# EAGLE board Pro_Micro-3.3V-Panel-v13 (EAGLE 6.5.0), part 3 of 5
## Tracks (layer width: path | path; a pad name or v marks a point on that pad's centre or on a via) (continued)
D223  (via drill 0.25)
  Top 0.203: U36.28 111.28,90.4 112.1,90.4 112.67,89.83 112.67,83.19 112.69,83.17 v112.69,81.78
  Bottom 0.203: JP70.2 102.44,81.46 112.37,81.46 v112.69,81.78
D224  (via drill 0.25)
  Top 0.203: 105.18,91.08 105,90.91 105,90.23 v104.75,89.98
  Bottom 0.203: v104.75,89.98 105.92,91.15 105.92,91.95 103.12,94.74 103.12,97.21 102.53,97.8 101.58,97.8 101.23,98.15 101.23,100.74 101.74,101.24 102.45,101.24 103.12,101.92 103.12,104.28 103.12,104.29 102.55,104.87 101.35,104.87 100.85,104.36 100.85,101.56 99.57,100.28 JP70.8
D225  (via drill 0.25)
  Top 0.203: 104.83,91.43 104.32,90.92 v104.29,90.92
  Bottom 0.203: JP70.7 100.84,95.76 100.84,93.98 101.35,93.47 101.35,92.08 102.5,90.92 v104.29,90.92
D226  (via drill 0.25)
  Top 0.203: 108.85,90.73 109.9,89.69 v109.9,89.28
  Bottom 0.203: JP70.6 100.84,93.22 100.84,91.24 101.22,90.86 101.22,88.47 101.71,87.97 101.71,85.78 102.19,85.31 107.23,85.31 108.88,86.97 108.88,87.62 109.9,88.64 v109.9,89.28
D227  (via drill 0.25)
  Top 0.203: 110.94,92.83 111.57,92.19 v111.93,92.19
  Bottom 0.203: JP70.5 100.84,90.68 100.84,88.9 100.8,88.86 100.8,88.28 101.29,87.78 101.29,85.58 102.06,84.82 107.35,84.82 109.3,86.76 109.3,87.38 109.31,87.38 110,88.07 110.55,88.07 111.16,88.68 111.16,89.21 110.41,89.96 109.43,89.96 109.14,90.25 109.14,91.08 109.71,91.65 111.38,91.65 v111.93,92.19
D228  (via drill 0.25)
  Top 0.203: v109.86,90.81 109.86,91.11 v109.86,90.81 | U36.27 109.86,91.12 v109.86,90.81
  Bottom 0.203: v109.86,90.81 110.31,90.81 111.67,89.44 111.67,88.54 110.79,87.67 110.17,87.67 109.71,87.21 109.71,86.54 107.47,84.3 101.83,84.3 100.81,85.32 100.81,87.59 99.57,88.83 JP70.4
D229  (via drill 0.25)
  Top 0.203: JP70.3 100.84,88.14 100.84,93.8 v101.53,94.49 | v102,104.1 102,104.06 102.21,103.84 102.21,103 102.47,102.73 104.24,102.73 104.49,102.98 104.96,102.98 105.39,102.55 105.39,101.96 105.14,101.71 105.14,101.03 105.33,100.85 107.01,100.85 107.01,100.83 107.39,100.45 108.02,100.45 108.12,100.34 108.12,99.59 107.54,99 106.84,99 106.54,99.3 106.36,99.3 106.22,99.16 106.22,98.94 U36.1 106.22,98.94
  Bottom 0.203: v102,104.1 101.96,104.1 101.3,103.44 101.3,101.41 100.84,100.95 100.84,96.65 101.53,95.96 v101.53,94.49
D230
  Top 0.203: JP69.12 114.81,82.47 113.56,83.72 113.56,90.22 112.54,91.24 111.83,91.24 U36.30
D234  (via drill 0.25)
  Top 0.203: R106.1 101.09,83.22 101.09,85.34 101.25,85.5 101.25,91.85 v102.01,92.62 | 103.79,96.49 103.25,97.03 v102.36,97.03
  Bottom 0.203: v102.36,97.03 102.36,92.97 v102.01,92.62
D+  (via drill 0.25)
  Top 0.203: v20.8,36.3 21.59,35.51 21.59,33.78 21.15,33.34 R5.1 | U3.4 13.58,24.39 13.58,26.18 v13.28,26.47
  Bottom 0.203: v20.8,36.3 20.95,36.14 20.95,29.94 19.31,28.3 19.31,26.73 17.77,25.2 17.77,25.18 14.57,25.18 v13.28,26.47
D+1  (via drill 0.25)
  Top 0.203: v39.09,36.3 39.88,35.51 39.88,33.78 39.44,33.34 R10.1 | U4.4 31.87,24.39 31.87,26.18 v31.57,26.47
  Bottom 0.203: v39.09,36.3 39.24,36.14 39.24,29.94 37.6,28.3 37.6,26.73 36.06,25.2 36.06,25.18 32.86,25.18 v31.57,26.47
D+2  (via drill 0.25)
  Top 0.203: v57.38,36.3 58.17,35.51 58.17,33.78 57.73,33.34 R17.1 | U6.4 50.16,24.39 50.16,26.18 v49.86,26.47
  Bottom 0.203: v57.38,36.3 57.53,36.14 57.53,29.94 55.88,28.3 55.88,26.73 54.35,25.2 54.35,25.18 51.15,25.18 v49.86,26.47
D+3  (via drill 0.25)
  Top 0.203: v75.67,36.3 76.45,35.51 76.45,33.78 76.02,33.34 R23.1 | U8.4 68.44,24.39 68.44,26.18 v68.15,26.47
  Bottom 0.203: v75.67,36.3 75.82,36.14 75.82,29.94 74.17,28.3 74.17,26.73 72.64,25.2 72.64,25.18 69.44,25.18 v68.15,26.47
D+4  (via drill 0.25)
  Top 0.203: v93.95,36.3 94.74,35.51 94.74,33.78 94.31,33.34 R29.1 | U10.4 86.73,24.39 86.73,26.18 v86.44,26.47
  Bottom 0.203: v93.95,36.3 94.11,36.14 94.11,29.94 92.46,28.3 92.46,26.73 90.92,25.2 90.92,25.18 87.73,25.18 v86.44,26.47
D+5  (via drill 0.25)
  Top 0.203: v112.24,36.3 113.03,35.51 113.03,33.78 112.59,33.34 R35.1 | U12.4 105.02,24.39 105.02,26.18 v104.72,26.47
  Bottom 0.203: v112.24,36.3 112.39,36.14 112.39,29.94 110.75,28.3 110.75,26.73 109.21,25.2 109.21,25.18 106.02,25.18 v104.72,26.47
D+6  (via drill 0.25)
  Top 0.203: v20.8,73.13 21.59,72.34 21.59,70.61 21.15,70.17 R41.1 | U14.4 13.58,61.22 13.58,63.01 v13.28,63.3
  Bottom 0.203: v20.8,73.13 20.95,72.97 20.95,66.77 19.31,65.13 19.31,63.56 17.77,62.03 17.77,62.01 14.57,62.01 v13.28,63.3
D+7  (via drill 0.25)
  Top 0.203: v39.09,73.13 39.88,72.34 39.88,70.61 39.44,70.17 R47.1 | U16.4 31.87,61.22 31.87,63.01 v31.57,63.3
  Bottom 0.203: v39.09,73.13 39.24,72.97 39.24,66.77 37.6,65.13 37.6,63.56 36.06,62.03 36.06,62.01 32.86,62.01 v31.57,63.3
D+8  (via drill 0.25)
  Top 0.203: v57.38,73.13 58.17,72.34 58.17,70.61 57.73,70.17 R53.1 | U18.4 50.16,61.22 50.16,63.01 v49.86,63.3
  Bottom 0.203: v57.38,73.13 57.53,72.97 57.53,66.77 55.88,65.13 55.88,63.56 54.35,62.03 54.35,62.01 51.15,62.01 v49.86,63.3
D+9  (via drill 0.25)
  Top 0.203: v75.67,73.13 76.45,72.34 76.45,70.61 76.02,70.17 R59.1 | U20.4 68.44,61.22 68.44,63.01 v68.15,63.3
  Bottom 0.203: v75.67,73.13 75.82,72.97 75.82,66.77 74.17,65.13 74.17,63.56 72.64,62.03 72.64,62.01 69.44,62.01 v68.15,63.3
D+10  (via drill 0.25)
  Top 0.203: v93.95,73.13 94.74,72.34 94.74,70.61 94.31,70.17 R65.1 | U22.4 86.73,61.22 86.73,63.01 v86.44,63.3
  Bottom 0.203: v93.95,73.13 94.11,72.97 94.11,66.77 92.46,65.13 92.46,63.56 90.92,62.03 90.92,62.01 87.73,62.01 v86.44,63.3
D+11  (via drill 0.25)
  Top 0.203: v112.24,73.13 113.03,72.34 113.03,70.61 112.59,70.17 R71.1 | U24.4 105.02,61.22 105.02,63.01 v104.72,63.3
  Bottom 0.203: v112.24,73.13 112.39,72.97 112.39,66.77 110.75,65.13 110.75,63.56 109.21,62.03 109.21,62.01 106.02,62.01 v104.72,63.3
D+12  (via drill 0.25)
  Top 0.203: v20.8,109.96 21.59,109.17 21.59,107.44 21.15,107 R77.1 | U26.4 13.58,98.05 13.58,99.83 v13.28,100.13
  Bottom 0.203: v20.8,109.96 20.95,109.8 20.95,103.6 19.31,101.96 19.31,100.39 17.77,98.86 17.77,98.84 14.57,98.84 v13.28,100.13
D+13  (via drill 0.25)
  Top 0.203: v39.09,109.96 39.88,109.17 39.88,107.44 39.44,107 R83.1 | U28.4 31.87,98.05 31.87,99.83 v31.57,100.13
  Bottom 0.203: v39.09,109.96 39.24,109.8 39.24,103.6 37.6,101.96 37.6,100.39 36.06,98.86 36.06,98.84 32.86,98.84 v31.57,100.13
D+14  (via drill 0.25)
  Top 0.203: v57.38,109.96 58.17,109.17 58.17,107.44 57.73,107 R89.1 | U30.4 50.16,98.05 50.16,99.83 v49.86,100.13
  Bottom 0.203: v57.38,109.96 57.53,109.8 57.53,103.6 55.88,101.96 55.88,100.39 54.35,98.86 54.35,98.84 51.15,98.84 v49.86,100.13
D+15  (via drill 0.25)
  Top 0.203: v75.67,109.96 76.45,109.17 76.45,107.44 76.02,107 R95.1 | U32.4 68.44,98.05 68.44,99.83 v68.15,100.13
  Bottom 0.203: v75.67,109.96 75.82,109.8 75.82,103.6 74.17,101.96 74.17,100.39 72.64,98.86 72.64,98.84 69.44,98.84 v68.15,100.13
D+16  (via drill 0.25)
  Top 0.203: v93.95,109.96 94.74,109.17 94.74,107.44 94.31,107 R101.1 | U34.4 86.73,98.05 86.73,99.83 v86.44,100.13
  Bottom 0.203: v93.95,109.96 94.11,109.8 94.11,103.6 92.46,101.96 92.46,100.39 90.92,98.86 90.92,98.84 87.73,98.84 v86.44,100.13
D+17  (via drill 0.25)
  Top 0.203: v112.24,109.96 113.03,109.17 113.03,107.44 112.59,107 R107.1 | U36.4 105.02,98.05 105.02,99.83 v104.72,100.13
  Bottom 0.203: v112.24,109.96 112.39,109.8 112.39,103.6 110.75,101.96 110.75,100.39 109.21,98.86 109.21,98.84 106.02,98.84 v104.72,100.13
D-  (via drill 0.25)
  Top 0.203: 20.41,35.12 R7.1 20.32,34.89 20.32,35.56 19.96,35.92 v19.96,37.08 | v14.25,26.5 13.99,26.25 13.99,24.67 14.1,24.57
  Bottom 0.203: v19.96,37.08 21.08,37.08 21.46,36.7 21.46,29.77 19.76,28.07 19.76,26.53 17.98,24.75 14.43,24.75 13.44,25.75 13.04,25.75 13.03,25.74 12.58,26.2 12.58,26.86 12.93,27.21 13.54,27.21 v14.25,26.5
D-1  (via drill 0.25)
  Top 0.203: 38.7,35.12 R12.1 38.61,34.89 38.61,35.56 38.25,35.92 v38.25,37.08 | v32.53,26.5 32.28,26.25 32.28,24.67 32.38,24.57
  Bottom 0.203: v38.25,37.08 39.37,37.08 39.75,36.7 39.75,29.77 38.05,28.07 38.05,26.53 36.27,24.75 32.72,24.75 31.73,25.75 31.33,25.75 31.32,25.74 30.87,26.2 30.87,26.86 31.22,27.21 31.83,27.21 v32.53,26.5
D-2  (via drill 0.25)
  Top 0.203: 56.98,35.12 R18.1 56.9,34.89 56.9,35.56 56.54,35.92 v56.54,37.08 | v50.82,26.5 50.57,26.25 50.57,24.67 50.67,24.57
  Bottom 0.203: v56.54,37.08 57.66,37.08 58.04,36.7 58.04,29.77 56.34,28.07 56.34,26.53 54.56,24.75 51.01,24.75 50.02,25.75 49.62,25.75 49.61,25.74 49.15,26.2 49.15,26.86 49.51,27.21 50.11,27.21 v50.82,26.5
D-3  (via drill 0.25)
  Top 0.203: 75.27,35.12 R24.1 75.18,34.89 75.18,35.56 74.83,35.92 v74.83,37.08 | v69.11,26.5 68.86,26.25 68.86,24.67 68.96,24.57
  Bottom 0.203: v74.83,37.08 75.95,37.08 76.33,36.7 76.33,29.77 74.62,28.07 74.62,26.53 72.85,24.75 69.3,24.75 68.3,25.75 67.9,25.75 67.9,25.74 67.44,26.2 67.44,26.86 67.79,27.21 68.4,27.21 v69.11,26.5
D-4  (via drill 0.25)
  Top 0.203: 93.56,35.12 R30.1 93.47,34.89 93.47,35.56 93.12,35.92 v93.12,37.08 | v87.4,26.5 87.15,26.25 87.15,24.67 87.25,24.57
  Bottom 0.203: v93.12,37.08 94.23,37.08 94.61,36.7 94.61,29.77 92.91,28.07 92.91,26.53 91.14,24.75 87.58,24.75 86.59,25.75 86.19,25.75 86.19,25.74 85.73,26.2 85.73,26.86 86.08,27.21 86.69,27.21 v87.4,26.5
D-5  (via drill 0.25)
  Top 0.203: 111.85,35.12 R36.1 111.76,34.89 111.76,35.56 111.4,35.92 v111.4,37.08 | v105.69,26.5 105.44,26.25 105.44,24.67 105.54,24.57
  Bottom 0.203: v111.4,37.08 112.52,37.08 112.9,36.7 112.9,29.77 111.2,28.07 111.2,26.53 109.42,24.75 105.87,24.75 104.88,25.75 104.48,25.75 104.47,25.74 104.02,26.2 104.02,26.86 104.37,27.21 104.98,27.21 v105.69,26.5
D-6  (via drill 0.25)
  Top 0.203: 20.41,71.95 R42.1 20.32,71.72 20.32,72.39 19.96,72.75 v19.96,73.91 | v14.25,63.34 13.99,63.08 13.99,61.5 14.1,61.4
  Bottom 0.203: v19.96,73.91 21.08,73.91 21.46,73.53 21.46,66.6 19.76,64.9 19.76,63.36 17.98,61.59 14.43,61.59 13.44,62.58 13.04,62.58 13.03,62.57 12.58,63.02 12.58,63.69 12.93,64.04 13.54,64.04 v14.25,63.34
D-7  (via drill 0.25)
  Top 0.203: 38.7,71.95 R48.1 38.61,71.72 38.61,72.39 38.25,72.75 v38.25,73.91 | v32.53,63.34 32.28,63.08 32.28,61.5 32.38,61.4
  Bottom 0.203: v38.25,73.91 39.37,73.91 39.75,73.53 39.75,66.6 38.05,64.9 38.05,63.36 36.27,61.59 32.72,61.59 31.73,62.58 31.33,62.58 31.32,62.57 30.87,63.02 30.87,63.69 31.22,64.04 31.83,64.04 v32.53,63.34
D-8  (via drill 0.25)
  Top 0.203: 56.98,71.95 R54.1 56.9,71.72 56.9,72.39 56.54,72.75 v56.54,73.91 | v50.82,63.34 50.57,63.08 50.57,61.5 50.67,61.4
  Bottom 0.203: v56.54,73.91 57.66,73.91 58.04,73.53 58.04,66.6 56.34,64.9 56.34,63.36 54.56,61.59 51.01,61.59 50.02,62.58 49.62,62.58 49.61,62.57 49.15,63.02 49.15,63.69 49.51,64.04 50.11,64.04 v50.82,63.34
D-9  (via drill 0.25)
  Top 0.203: 75.27,71.95 R60.1 75.18,71.72 75.18,72.39 74.83,72.75 v74.83,73.91 | v69.11,63.34 68.86,63.08 68.86,61.5 68.96,61.4
  Bottom 0.203: v74.83,73.91 75.95,73.91 76.33,73.53 76.33,66.6 74.62,64.9 74.62,63.36 72.85,61.59 69.3,61.59 68.3,62.58 67.9,62.58 67.9,62.57 67.44,63.02 67.44,63.69 67.79,64.04 68.4,64.04 v69.11,63.34
D-10  (via drill 0.25)
  Top 0.203: 93.56,71.95 R66.1 93.47,71.72 93.47,72.39 93.12,72.75 v93.12,73.91 | v87.4,63.34 87.15,63.08 87.15,61.5 87.25,61.4
  Bottom 0.203: v93.12,73.91 94.23,73.91 94.61,73.53 94.61,66.6 92.91,64.9 92.91,63.36 91.14,61.59 87.58,61.59 86.59,62.58 86.19,62.58 86.19,62.57 85.73,63.02 85.73,63.69 86.08,64.04 86.69,64.04 v87.4,63.34
D-11  (via drill 0.25)
  Top 0.203: 111.85,71.95 R72.1 111.76,71.72 111.76,72.39 111.4,72.75 v111.4,73.91 | v105.69,63.34 105.44,63.08 105.44,61.5 105.54,61.4
  Bottom 0.203: v111.4,73.91 112.52,73.91 112.9,73.53 112.9,66.6 111.2,64.9 111.2,63.36 109.42,61.59 105.87,61.59 104.88,62.58 104.48,62.58 104.47,62.57 104.02,63.02 104.02,63.69 104.37,64.04 104.98,64.04 v105.69,63.34
D-12  (via drill 0.25)
  Top 0.203: 20.41,108.78 R78.1 20.32,108.55 20.32,109.22 19.96,109.58 v19.96,110.74 | v14.25,100.17 13.99,99.91 13.99,98.33 14.1,98.23
  Bottom 0.203: v19.96,110.74 21.08,110.74 21.46,110.36 21.46,103.43 19.76,101.73 19.76,100.19 17.98,98.42 14.43,98.42 13.44,99.41 13.04,99.41 13.03,99.4 12.58,99.86 12.58,100.52 12.93,100.87 13.54,100.87 v14.25,100.17
D-13  (via drill 0.25)
  Top 0.203: 38.7,108.78 R84.1 38.61,108.55 38.61,109.22 38.25,109.58 v38.25,110.74 | v32.53,100.17 32.28,99.91 32.28,98.33 32.38,98.23
  Bottom 0.203: v38.25,110.74 39.37,110.74 39.75,110.36 39.75,103.43 38.05,101.73 38.05,100.19 36.27,98.42 32.72,98.42 31.73,99.41 31.33,99.41 31.32,99.4 30.87,99.86 30.87,100.52 31.22,100.87 31.83,100.87 v32.53,100.17
D-14  (via drill 0.25)
  Top 0.203: 56.98,108.78 R90.1 56.9,108.55 56.9,109.22 56.54,109.58 v56.54,110.74 | v50.82,100.17 50.57,99.91 50.57,98.33 50.67,98.23
  Bottom 0.203: v56.54,110.74 57.66,110.74 58.04,110.36 58.04,103.43 56.34,101.73 56.34,100.19 54.56,98.42 51.01,98.42 50.02,99.41 49.62,99.41 49.61,99.4 49.15,99.86 49.15,100.52 49.51,100.87 50.11,100.87 v50.82,100.17
D-15  (via drill 0.25)
  Top 0.203: 75.27,108.78 R96.1 75.18,108.55 75.18,109.22 74.83,109.58 v74.83,110.74 | v69.11,100.17 68.86,99.91 68.86,98.33 68.96,98.23
  Bottom 0.203: v74.83,110.74 75.95,110.74 76.33,110.36 76.33,103.43 74.62,101.73 74.62,100.19 72.85,98.42 69.3,98.42 68.3,99.41 67.9,99.41 67.9,99.4 67.44,99.86 67.44,100.52 67.79,100.87 68.4,100.87 v69.11,100.17
D-16  (via drill 0.25)
  Top 0.203: 93.56,108.78 R102.1 93.47,108.55 93.47,109.22 93.12,109.58 v93.12,110.74 | v87.4,100.17 87.15,99.91 87.15,98.33 87.25,98.23
  Bottom 0.203: v93.12,110.74 94.23,110.74 94.61,110.36 94.61,103.43 92.91,101.73 92.91,100.19 91.14,98.42 87.58,98.42 86.59,99.41 86.19,99.41 86.19,99.4 85.73,99.86 85.73,100.52 86.08,100.87 86.69,100.87 v87.4,100.17
D-17  (via drill 0.25)
  Top 0.203: 111.85,108.78 R108.1 111.76,108.55 111.76,109.22 111.4,109.58 v111.4,110.74 | v105.69,100.17 105.44,99.91 105.44,98.33 105.54,98.23
  Bottom 0.203: v111.4,110.74 112.52,110.74 112.9,110.36 112.9,103.43 111.2,101.73 111.2,100.19 109.42,98.42 105.87,98.42 104.88,99.41 104.48,99.41 104.47,99.4 104.02,99.86 104.02,100.52 104.37,100.87 104.98,100.87 v105.69,100.17
GND  (via drill 0.25)
  Top 0.203: v20.57,19.48 | U3.33 20.5,19.56 20.83,19.56 | C3.1 20.07,14.33 | 12.34,18.82 12.22,18.82 11.76,18.36 11.52,18.36 11.05,17.89 11.05,17.32 11.32,17.06 C10.2 11.49,15.41 12.12,14.78 12.12,13.64 12.99,12.77 C4.2 | 16.71,16.38 16.76,16.33 16.76,15.93 | 18.2,13.84 arc-21 v19.05,13.31 | 12.24,27.31 C13.C 12.56,26.67 C5.1 12.56,24.71 13.4,23.87
  Top 0.406: X1.GND1 14.45,37.34 14.48,37.34
  Bottom 0.203: JP7.10 9.25,32.11 v10.2,32.11
  other vias: 15.99,9.86 21.72,25.53 18.76,28.77 20.74,22.7 17.74,26.5 13.25,28.57 23.94,38.23 15.44,32.56 22.26,29.71 13.68,37.82 10.37,9.85 12.46,13.81 13.28,31.04 16.41,13.92
  pour Top (isolate 0.203): 6.86,39.88 24.64,39.88 24.64,6.86 6.86,6.86
  pour Bottom (isolate 0.203): 6.86,39.88 24.64,39.88 24.64,6.86 6.86,6.86
GND1  (via drill 0.25)
  Top 0.203: v38.86,19.48 | U4.33 38.79,19.56 39.12,19.56 | C9.1 38.35,14.33 | 30.63,18.82 30.51,18.82 30.05,18.36 29.81,18.36 29.34,17.89 29.34,17.32 29.6,17.06 C7.2 29.78,15.41 30.41,14.78 30.41,13.64 31.28,12.77 C15.2 | 35,16.38 35.05,16.33 35.05,15.93 | 36.49,13.84 arc-21 v37.33,13.31 | 30.53,27.31 C8.C 30.85,26.67 C16.1 30.85,24.71 31.69,23.87
  Top 0.406: X2.GND1 32.74,37.34 32.77,37.34
  Bottom 0.203: JP4.10 27.54,32.11 v28.49,32.11
  other vias: 34.27,9.86 40.01,25.53 37.05,28.77 39.03,22.7 36.03,26.5 31.54,28.57 42.23,38.23 33.73,32.56 40.54,29.71 31.97,37.82 28.65,9.85 30.75,13.81 31.57,31.04 34.7,13.92
  pour Top (isolate 0.203): 25.15,39.88 42.93,39.88 42.93,6.86 25.15,6.86
  pour Bottom (isolate 0.203): 25.15,39.88 42.93,39.88 42.93,6.86 25.15,6.86
GND2  (via drill 0.25)
  Top 0.203: v57.15,19.48 | U6.33 57.08,19.56 57.4,19.56 | C21.1 56.64,14.33 | 48.92,18.82 48.79,18.82 48.33,18.36 48.09,18.36 47.63,17.89 47.63,17.32 47.89,17.06 C18.2 48.06,15.41 48.07,15.41 48.7,14.78 48.7,13.64 49.57,12.77 C25.2 | 53.29,16.38 53.34,16.33 53.34,15.93 | 54.77,13.84 arc-21 v55.62,13.31 | 48.81,27.31 C20.C 49.14,26.67 C26.1 49.14,24.71 49.98,23.87
  Top 0.406: X3.GND1 51.02,37.34 51.05,37.34
  Bottom 0.203: JP10.10 45.83,32.11 v46.77,32.11
  other vias: 52.56,9.86 58.29,25.53 55.34,28.77 57.32,22.7 54.32,26.5 49.82,28.57 60.52,38.23 52.02,32.56 58.83,29.71 50.25,37.82 46.94,9.85 49.03,13.81 49.86,31.04 52.99,13.92
  pour Top (isolate 0.203): 43.43,39.88 61.21,39.88 61.21,6.86 43.43,6.86
  pour Bottom (isolate 0.203): 43.43,39.88 61.21,39.88 61.21,6.86 43.43,6.86
GND3  (via drill 0.25)
  Top 0.203: v75.43,19.48 v75.44,19.48 | U8.33 75.37,19.56 75.69,19.56 | C30.1 74.93,14.33 | 67.21,18.82 67.08,18.82 66.62,18.36 66.38,18.36 65.92,17.89 65.92,17.32 66.18,17.06 C28.2 66.35,15.41 66.36,15.41 66.98,14.78 66.98,13.64 67.86,12.77 C34.2 | 71.58,16.38 71.63,16.33 71.63,15.93 | 73.06,13.84 arc-21 v73.91,13.31 | 67.1,27.31 C29.C 67.43,26.67 C35.1 67.43,24.71 68.26,23.87
  Top 0.406: X4.GND1 69.31,37.34 69.34,37.34
  Bottom 0.203: JP14.10 64.11,32.11 v65.06,32.11
  other vias: 70.85,9.86 76.58,25.53 73.62,28.77 75.6,22.7 72.61,26.5 68.11,28.57 78.8,38.23 70.3,32.56 77.12,29.71 68.54,37.82 65.23,9.85 67.32,13.81 68.15,31.04 71.28,13.92
  pour Top (isolate 0.203): 61.72,39.88 79.5,39.88 79.5,6.86 61.72,6.86
  pour Bottom (isolate 0.203): 61.72,39.88 79.5,39.88 79.5,6.86 61.72,6.86
GND4  (via drill 0.25)
  Top 0.203: v93.72,19.48 v93.73,19.48 | U10.33 93.66,19.56 93.98,19.56 | C39.1 93.22,14.33 | 85.5,18.82 85.37,18.82 84.91,18.36 84.67,18.36 84.21,17.89 84.21,17.32 84.47,17.06 C37.2 84.64,15.41 85.27,14.78 85.27,13.64 86.14,12.77 C43.2 | 89.86,16.38 89.92,16.33 89.92,15.93 | 91.35,13.84 arc-21 v92.2,13.31 | 85.39,27.31 C38.C 85.71,26.67 C44.1 85.71,24.71 86.55,23.87
  Top 0.406: X5.GND1 87.6,37.34 87.63,37.34
  Bottom 0.203: JP18.10 82.4,32.11 v83.35,32.11
  other vias: 89.14,9.86 94.87,25.53 91.91,28.77 93.89,22.7 90.89,26.5 86.4,28.57 97.09,38.23 88.59,32.56 95.41,29.71 86.83,37.82 83.52,9.85 85.61,13.81 86.44,31.04 89.57,13.92
  pour Top (isolate 0.203): 80.01,39.88 97.79,39.88 97.79,6.86 80.01,6.86
  pour Bottom (isolate 0.203): 80.01,39.88 97.79,39.88 97.79,6.86 80.01,6.86
GND5  (via drill 0.25)
  Top 0.203: v112.01,19.48 | U12.33 111.94,19.56 112.27,19.56 | C48.1 111.51,14.33 | 103.78,18.82 103.66,18.82 103.2,18.36 102.96,18.36 102.49,17.89 102.49,17.32 102.76,17.06 C46.2 102.93,15.41 103.56,14.78 103.56,13.64 104.43,12.77 C52.2 | 108.15,16.38 108.2,16.33 108.2,15.93 | 109.64,13.84 arc-21 v110.48,13.31 | 103.68,27.31 C47.C 104,26.67 C53.1 104,24.71 104.84,23.87
  Top 0.406: X6.GND1 105.89,37.34 105.92,37.34
  Bottom 0.203: JP22.10 100.69,32.11 v101.64,32.11
  other vias: 107.43,9.86 113.16,25.53 110.2,28.77 112.18,22.7 109.18,26.5 104.69,28.57 115.38,38.23 106.88,32.56 113.7,29.71 105.12,37.82 101.81,9.85 103.9,13.81 104.72,31.04 107.85,13.92
  pour Top (isolate 0.203): 98.3,39.88 116.08,39.88 116.08,6.86 98.3,6.86
  pour Bottom (isolate 0.203): 98.3,39.88 116.08,39.88 116.08,6.86 98.3,6.86
GND6  (via drill 0.25)
  Top 0.203: v20.57,56.31 | U14.33 20.5,56.39 20.83,56.39 | C57.1 20.07,51.16 | 12.34,55.65 12.22,55.65 11.76,55.19 11.52,55.19 11.05,54.72 11.05,54.15 11.32,53.89 C55.2 11.49,52.24 12.12,51.61 12.12,50.47 12.99,49.59 C61.2 | 16.71,53.21 16.76,53.16 16.76,52.76 | 18.2,50.67 arc-21 v19.05,50.15 | 12.24,64.14 C56.C 12.56,63.5 C62.1 12.56,61.54 13.4,60.7
  Top 0.406: X7.GND1 14.45,74.17 14.48,74.17
  Bottom 0.203: JP26.10 9.25,68.94 v10.2,68.94
  other vias: 15.99,46.69 21.72,62.36 18.76,65.6 20.74,59.53 17.74,63.33 13.25,65.4 23.94,75.06 15.44,69.39 22.26,66.54 13.68,74.65 10.37,46.68 12.46,50.64 13.28,67.87 16.41,50.75
  pour Top (isolate 0.203): 6.86,76.71 24.64,76.71 24.64,43.69 6.86,43.69
  pour Bottom (isolate 0.203): 6.86,76.71 24.64,76.71 24.64,43.69 6.86,43.69
GND7  (via drill 0.25)
  Top 0.203: v38.86,56.31 | U16.33 38.79,56.39 39.12,56.39 | C66.1 38.35,51.16 | 30.63,55.65 30.51,55.65 30.05,55.19 29.81,55.19 29.34,54.72 29.34,54.15 29.6,53.89 C64.2 29.78,52.24 30.41,51.61 30.41,50.47 31.28,49.59 C70.2 | 35,53.21 35.05,53.16 35.05,52.76 | 36.49,50.67 arc-21 v37.33,50.15 | 30.53,64.14 C65.C 30.85,63.5 C71.1 30.85,61.54 31.69,60.7
  Top 0.406: X8.GND1 32.74,74.17 32.77,74.17
  Bottom 0.203: JP30.10 27.54,68.94 v28.49,68.94
  other vias: 34.27,46.69 40.01,62.36 37.05,65.6 39.03,59.53 36.03,63.33 31.54,65.4 42.23,75.06 33.73,69.39 40.54,66.54 31.97,74.65 28.65,46.68 30.75,50.64 31.57,67.87 34.7,50.75
  pour Top (isolate 0.203): 25.15,76.71 42.93,76.71 42.93,43.69 25.15,43.69
  pour Bottom (isolate 0.203): 25.15,76.71 42.93,76.71 42.93,43.69 25.15,43.69
GND8  (via drill 0.25)
  Top 0.203: v57.15,56.31 | U18.33 57.08,56.39 57.4,56.39 | C75.1 56.64,51.16 | 48.92,55.65 48.79,55.65 48.33,55.19 48.09,55.19 47.63,54.72 47.63,54.15 47.89,53.89 C73.2 48.06,52.24 48.07,52.24 48.7,51.61 48.7,50.47 49.57,49.59 C79.2 | 53.29,53.21 53.34,53.16 53.34,52.76 | 54.77,50.67 arc-21 v55.62,50.15 | 48.81,64.14 C74.C 49.14,63.5 C80.1 49.14,61.54 49.98,60.7
  Top 0.406: X9.GND1 51.02,74.17 51.05,74.17
  Bottom 0.203: JP34.10 45.83,68.94 v46.77,68.94
  other vias: 52.56,46.69 58.29,62.36 55.34,65.6 57.32,59.53 54.32,63.33 49.82,65.4 60.52,75.06 52.02,69.39 58.83,66.54 50.25,74.65 46.94,46.68 49.03,50.64 49.86,67.87 52.99,50.75
  pour Top (isolate 0.203): 43.43,76.71 61.21,76.71 61.21,43.69 43.43,43.69
  pour Bottom (isolate 0.203): 43.43,76.71 61.21,76.71 61.21,43.69 43.43,43.69
GND9  (via drill 0.25)
  Top 0.203: v75.43,56.31 v75.44,56.31 | U20.33 75.37,56.39 75.69,56.39 | C84.1 74.93,51.16 | 67.21,55.65 67.08,55.65 66.62,55.19 66.38,55.19 65.92,54.72 65.92,54.15 66.18,53.89 C82.2 66.35,52.24 66.36,52.24 66.98,51.61 66.98,50.47 67.86,49.59 C88.2 | 71.58,53.21 71.63,53.16 71.63,52.76 | 73.06,50.67 arc-21 v73.91,50.15 | 67.1,64.14 C83.C 67.43,63.5 C89.1 67.43,61.54 68.26,60.7
  Top 0.406: X10.GND1 69.31,74.17 69.34,74.17
  Bottom 0.203: JP38.10 64.11,68.94 v65.06,68.94
  other vias: 70.85,46.69 76.58,62.36 73.62,65.6 75.6,59.53 72.61,63.33 68.11,65.4 78.8,75.06 70.3,69.39 77.12,66.54 68.54,74.65 65.23,46.68 67.32,50.64 68.15,67.87 71.28,50.75
  pour Top (isolate 0.203): 61.72,76.71 79.5,76.71 79.5,43.69 61.72,43.69
  pour Bottom (isolate 0.203): 61.72,76.71 79.5,76.71 79.5,43.69 61.72,43.69
GND10  (via drill 0.25)
  Top 0.203: v93.72,56.31 v93.73,56.31 | U22.33 93.66,56.39 93.98,56.39 | C93.1 93.22,51.16 | 85.5,55.65 85.37,55.65 84.91,55.19 84.67,55.19 84.21,54.72 84.21,54.15 84.47,53.89 C91.2 84.64,52.24 85.27,51.61 85.27,50.47 86.14,49.59 C97.2 | 89.86,53.21 89.92,53.16 89.92,52.76 | 91.35,50.67 arc-21 v92.2,50.15 | 85.39,64.14 C92.C 85.71,63.5 C98.1 85.71,61.54 86.55,60.7
  Top 0.406: X11.GND1 87.6,74.17 87.63,74.17
  Bottom 0.203: JP42.10 82.4,68.94 v83.35,68.94
  other vias: 89.14,46.69 94.87,62.36 91.91,65.6 93.89,59.53 90.89,63.33 86.4,65.4 97.09,75.06 88.59,69.39 95.41,66.54 86.83,74.65 83.52,46.68 85.61,50.64 86.44,67.87 89.57,50.75
  pour Top (isolate 0.203): 80.01,76.71 97.79,76.71 97.79,43.69 80.01,43.69
  pour Bottom (isolate 0.203): 80.01,76.71 97.79,76.71 97.79,43.69 80.01,43.69
GND11  (via drill 0.25)
  Top 0.203: v112.01,56.31 | U24.33 111.94,56.39 112.27,56.39 | C102.1 111.51,51.16 | 103.78,55.65 103.66,55.65 103.2,55.19 102.96,55.19 102.49,54.72 102.49,54.15 102.76,53.89 C100.2 102.93,52.24 103.56,51.61 103.56,50.47 104.43,49.59 C106.2 | 108.15,53.21 108.2,53.16 108.2,52.76 | 109.64,50.67 arc-21 v110.48,50.15 | 103.68,64.14 C101.C 104,63.5 C107.1 104,61.54 104.84,60.7
  Top 0.406: X12.GND1 105.89,74.17 105.92,74.17
  Bottom 0.203: JP46.10 100.69,68.94 v101.64,68.94
  other vias: 107.43,46.69 113.16,62.36 110.2,65.6 112.18,59.53 109.18,63.33 104.69,65.4 115.38,75.06 106.88,69.39 113.7,66.54 105.12,74.65 101.81,46.68 103.9,50.64 104.72,67.87 107.85,50.75
  pour Top (isolate 0.203): 98.3,76.71 116.08,76.71 116.08,43.69 98.3,43.69
  pour Bottom (isolate 0.203): 98.3,76.71 116.08,76.71 116.08,43.69 98.3,43.69
GND12  (via drill 0.25)
  Top 0.203: v20.57,93.14 | U26.33 20.5,93.22 20.83,93.22 | C111.1 20.07,87.99 | 12.34,92.48 12.22,92.48 11.76,92.02 11.52,92.02 11.05,91.55 11.05,90.98 11.32,90.72 C109.2 11.49,89.07 12.12,88.44 12.12,87.3 12.99,86.42 C115.2 | 16.71,90.04 16.76,89.99 16.76,89.59 | 18.2,87.5 arc-21 v19.05,86.97 | 12.24,100.97 C110.C 12.56,100.33 C116.1 12.56,98.37 13.4,97.53
  Top 0.406: X13.GND1 14.45,111 14.48,111
  Bottom 0.203: JP50.10 9.25,105.77 v10.2,105.77
  other vias: 15.99,83.52 21.72,99.19 18.76,102.43 20.74,96.36 17.74,100.16 13.25,102.23 23.94,111.89 15.44,106.22 22.26,103.37 13.68,111.48 10.37,83.51 12.46,87.47 13.28,104.7 16.41,87.58
  pour Top (isolate 0.203): 6.86,113.54 24.64,113.54 24.64,80.52 6.86,80.52
  pour Bottom (isolate 0.203): 6.86,113.54 24.64,113.54 24.64,80.52 6.86,80.52
GND13  (via drill 0.25)
  Top 0.203: v38.86,93.14 | U28.33 38.79,93.22 39.12,93.22 | C120.1 38.35,87.99 | 30.63,92.48 30.51,92.48 30.05,92.02 29.81,92.02 29.34,91.55 29.34,90.98 29.6,90.72 C118.2 29.78,89.07 30.41,88.44 30.41,87.3 31.28,86.42 C124.2 | 35,90.04 35.05,89.99 35.05,89.59 | 36.49,87.5 arc-21 v37.33,86.97 | 30.53,100.97 C119.C 30.85,100.33 C125.1 30.85,98.37 31.69,97.53
  Top 0.406: X14.GND1 32.74,111 32.77,111
  Bottom 0.203: JP54.10 27.54,105.77 v28.49,105.77
  other vias: 34.27,83.52 40.01,99.19 37.05,102.43 39.03,96.36 36.03,100.16 31.54,102.23 42.23,111.89 33.73,106.22 40.54,103.37 31.97,111.48 28.65,83.51 30.75,87.47 31.57,104.7 34.7,87.58
  pour Top (isolate 0.203): 25.15,113.54 42.93,113.54 42.93,80.52 25.15,80.52
  pour Bottom (isolate 0.203): 25.15,113.54 42.93,113.54 42.93,80.52 25.15,80.52
GND14  (via drill 0.25)
  Top 0.203: v57.15,93.14 | U30.33 57.08,93.22 57.4,93.22 | C129.1 56.64,87.99 | 48.92,92.48 48.79,92.48 48.33,92.02 48.09,92.02 47.63,91.55 47.63,90.98 47.89,90.72 C127.2 48.06,89.07 48.07,89.07 48.7,88.44 48.7,87.3 49.57,86.42 C133.2 | 53.29,90.04 53.34,89.99 53.34,89.59 | 54.77,87.5 arc-21 v55.62,86.97 | 48.81,100.97 C128.C 49.14,100.33 C134.1 49.14,98.37 49.98,97.53
  Top 0.406: X15.GND1 51.02,111 51.05,111
  Bottom 0.203: JP58.10 45.83,105.77 v46.77,105.77
  other vias: 52.56,83.52 58.29,99.19 55.34,102.43 57.32,96.36 54.32,100.16 49.82,102.23 60.52,111.89 52.02,106.22 58.83,103.37 50.25,111.48 46.94,83.51 49.03,87.47 49.86,104.7 52.99,87.58
  pour Top (isolate 0.203): 43.43,113.54 61.21,113.54 61.21,80.52 43.43,80.52
  pour Bottom (isolate 0.203): 43.43,113.54 61.21,113.54 61.21,80.52 43.43,80.52
GND15  (via drill 0.25)
  Top 0.203: v75.43,93.14 v75.44,93.14 | U32.33 75.37,93.22 75.69,93.22 | C138.1 74.93,87.99 | 67.21,92.48 67.08,92.48 66.62,92.02 66.38,92.02 65.92,91.55 65.92,90.98 66.18,90.72 C136.2 66.35,89.07 66.36,89.07 66.98,88.44 66.98,87.3 67.86,86.42 C142.2 | 71.58,90.04 71.63,89.99 71.63,89.59 | 73.06,87.5 arc-21 v73.91,86.97 | 67.1,100.97 C137.C 67.43,100.33 C143.1 67.43,98.37 68.26,97.53
  Top 0.406: X16.GND1 69.31,111 69.34,111
  Bottom 0.203: JP62.10 64.11,105.77 v65.06,105.77
  other vias: 70.85,83.52 76.58,99.19 73.62,102.43 75.6,96.36 72.61,100.16 68.11,102.23 78.8,111.89 70.3,106.22 77.12,103.37 68.54,111.48 65.23,83.51 67.32,87.47 68.15,104.7 71.28,87.58
  pour Top (isolate 0.203): 61.72,113.54 79.5,113.54 79.5,80.52 61.72,80.52
  pour Bottom (isolate 0.203): 61.72,113.54 79.5,113.54 79.5,80.52 61.72,80.52
GND16  (via drill 0.25)
  Top 0.203: v93.72,93.14 v93.73,93.14 | U34.33 93.66,93.22 93.98,93.22 | C147.1 93.22,87.99 | 85.5,92.48 85.37,92.48 84.91,92.02 84.67,92.02 84.21,91.55 84.21,90.98 84.47,90.72 C145.2 84.64,89.07 85.27,88.44 85.27,87.3 86.14,86.42 C151.2 | 89.86,90.04 89.92,89.99 89.92,89.59 | 91.35,87.5 arc-21 v92.2,86.97 | 85.39,100.97 C146.C 85.71,100.33 C152.1 85.71,98.37 86.55,97.53
  Top 0.406: X17.GND1 87.6,111 87.63,111
  Bottom 0.203: JP66.10 82.4,105.77 v83.35,105.77
  other vias: 89.14,83.52 94.87,99.19 91.91,102.43 93.89,96.36 90.89,100.16 86.4,102.23 97.09,111.89 88.59,106.22 95.41,103.37 86.83,111.48 83.52,83.51 85.61,87.47 86.44,104.7 89.57,87.58
  pour Top (isolate 0.203): 80.01,113.54 97.79,113.54 97.79,80.52 80.01,80.52
  pour Bottom (isolate 0.203): 80.01,113.54 97.79,113.54 97.79,80.52 80.01,80.52
GND17  (via drill 0.25)
  Top 0.203: v112.01,93.14 | U36.33 111.94,93.22 112.27,93.22 | C156.1 111.51,87.99 | 103.78,92.48 103.66,92.48 103.2,92.02 102.96,92.02 102.49,91.55 102.49,90.98 102.76,90.72 C154.2 102.93,89.07 103.56,88.44 103.56,87.3 104.43,86.42 C160.2 | 108.15,90.04 108.2,89.99 108.2,89.59 | 109.64,87.5 arc-21 v110.48,86.97 | 103.68,100.97 C155.C 104,100.33 C161.1 104,98.37 104.84,97.53
  Top 0.406: X18.GND1 105.89,111 105.92,111
  Bottom 0.203: JP70.10 100.69,105.77 v101.64,105.77
  other vias: 107.43,83.52 113.16,99.19 110.2,102.43 112.18,96.36 109.18,100.16 104.69,102.23 115.38,111.89 106.88,106.22 113.7,103.37 105.12,111.48 101.81,83.51 103.9,87.47 104.72,104.7 107.85,87.58
  pour Top (isolate 0.203): 98.3,113.54 116.08,113.54 116.08,80.52 98.3,80.52
  pour Bottom (isolate 0.203): 98.3,113.54 116.08,113.54 116.08,80.52 98.3,80.52
MISO  (via drill 0.25)
  Top 0.203: v16.82,21.11 16.03,20.32 14.61,20.32 14.1,20.83 12.26,20.83 U3.11
  Bottom 0.203: JP6.10 23.29,13.21 21.67,14.83 21.67,20.27 21.26,20.68 20.73,20.68 20.32,21.08 16.84,21.08 v16.82,21.11
MISO1  (via drill 0.25)
  Top 0.203: v35.1,21.11 34.31,20.32 32.89,20.32 32.38,20.83 30.55,20.83 U4.11
  Bottom 0.203: JP3.10 41.58,13.21 39.95,14.83 39.95,20.27 39.55,20.68 39.01,20.68 38.61,21.08 35.13,21.08 v35.1,21.11
MISO2  (via drill 0.25)
  Top 0.203: v53.39,21.11 52.6,20.32 51.18,20.32 50.67,20.83 48.84,20.83 U6.11
  Bottom 0.203: JP9.10 59.87,13.21 58.24,14.83 58.24,20.27 57.84,20.68 57.3,20.68 56.9,21.08 53.42,21.08 v53.39,21.11
MISO3  (via drill 0.25)
  Top 0.203: v71.68,21.11 70.89,20.32 69.47,20.32 68.96,20.83 67.13,20.83 U8.11
  Bottom 0.203: JP13.10 78.16,13.21 76.53,14.83 76.53,20.27 76.12,20.68 75.59,20.68 75.18,21.08 71.7,21.08 v71.68,21.11
MISO4  (via drill 0.25)
  Top 0.203: v89.97,21.11 89.18,20.32 87.76,20.32 87.25,20.83 85.41,20.83 U10.11
  Bottom 0.203: JP17.10 96.44,13.21 94.82,14.83 94.82,20.27 94.41,20.68 93.88,20.68 93.47,21.08 89.99,21.08 v89.97,21.11
MISO5  (via drill 0.25)
  Top 0.203: v108.25,21.11 107.47,20.32 106.05,20.32 105.54,20.83 103.7,20.83 U12.11
  Bottom 0.203: JP21.10 114.73,13.21 113.11,14.83 113.11,20.27 112.7,20.68 112.17,20.68 111.76,21.08 108.28,21.08 v108.25,21.11
MISO6  (via drill 0.25)
  Top 0.203: v16.82,57.94 16.03,57.15 14.61,57.15 14.1,57.66 12.26,57.66 U14.11
  Bottom 0.203: JP25.10 23.29,50.04 21.67,51.66 21.67,57.1 21.26,57.51 20.73,57.51 20.32,57.91 16.84,57.91 v16.82,57.94
MISO7  (via drill 0.25)
  Top 0.203: v35.1,57.94 34.31,57.15 32.89,57.15 32.38,57.66 30.55,57.66 U16.11
  Bottom 0.203: JP29.10 41.58,50.04 39.95,51.66 39.95,57.1 39.55,57.51 39.01,57.51 38.61,57.91 35.13,57.91 v35.1,57.94
MISO8  (via drill 0.25)
  Top 0.203: v53.39,57.94 52.6,57.15 51.18,57.15 50.67,57.66 48.84,57.66 U18.11
  Bottom 0.203: JP33.10 59.87,50.04 58.24,51.66 58.24,57.1 57.84,57.51 57.3,57.51 56.9,57.91 53.42,57.91 v53.39,57.94
MISO9  (via drill 0.25)
  Top 0.203: v71.68,57.94 70.89,57.15 69.47,57.15 68.96,57.66 67.13,57.66 U20.11
  Bottom 0.203: JP37.10 78.16,50.04 76.53,51.66 76.53,57.1 76.12,57.51 75.59,57.51 75.18,57.91 71.7,57.91 v71.68,57.94
MISO10  (via drill 0.25)
  Top 0.203: v89.97,57.94 89.18,57.15 87.76,57.15 87.25,57.66 85.41,57.66 U22.11
  Bottom 0.203: JP41.10 96.44,50.04 94.82,51.66 94.82,57.1 94.41,57.51 93.88,57.51 93.47,57.91 89.99,57.91 v89.97,57.94
MISO11  (via drill 0.25)
  Top 0.203: v108.25,57.94 107.47,57.15 106.05,57.15 105.54,57.66 103.7,57.66 U24.11
  Bottom 0.203: JP45.10 114.73,50.04 113.11,51.66 113.11,57.1 112.7,57.51 112.17,57.51 111.76,57.91 108.28,57.91 v108.25,57.94
MISO12  (via drill 0.25)
  Top 0.203: v16.82,94.77 16.03,93.98 14.61,93.98 14.1,94.49 12.26,94.49 U26.11
  Bottom 0.203: JP49.10 23.29,86.87 21.67,88.49 21.67,93.93 21.26,94.34 20.73,94.34 20.32,94.74 16.84,94.74 v16.82,94.77
MISO13  (via drill 0.25)
  Top 0.203: v35.1,94.77 34.31,93.98 32.89,93.98 32.38,94.49 30.55,94.49 U28.11
  Bottom 0.203: JP53.10 41.58,86.87 39.95,88.49 39.95,93.93 39.55,94.34 39.01,94.34 38.61,94.74 35.13,94.74 v35.1,94.77
MISO14  (via drill 0.25)
  Top 0.203: v53.39,94.77 52.6,93.98 51.18,93.98 50.67,94.49 48.84,94.49 U30.11
  Bottom 0.203: JP57.10 59.87,86.87 58.24,88.49 58.24,93.93 57.84,94.34 57.3,94.34 56.9,94.74 53.42,94.74 v53.39,94.77
MISO15  (via drill 0.25)
  Top 0.203: v71.68,94.77 70.89,93.98 69.47,93.98 68.96,94.49 67.13,94.49 U32.11
  Bottom 0.203: JP61.10 78.16,86.87 76.53,88.49 76.53,93.93 76.12,94.34 75.59,94.34 75.18,94.74 71.7,94.74 v71.68,94.77
MISO16  (via drill 0.25)
  Top 0.203: v89.97,94.77 89.18,93.98 87.76,93.98 87.25,94.49 85.41,94.49 U34.11
  Bottom 0.203: JP65.10 96.44,86.87 94.82,88.49 94.82,93.93 94.41,94.34 93.88,94.34 93.47,94.74 89.99,94.74 v89.97,94.77
MISO17  (via drill 0.25)
  Top 0.203: v108.25,94.77 107.47,93.98 106.05,93.98 105.54,94.49 103.7,94.49 U36.11
  Bottom 0.203: JP69.10 114.73,86.87 113.11,88.49 113.11,93.93 112.7,94.34 112.17,94.34 111.76,94.74 108.28,94.74 v108.25,94.77
MOSI  (via drill 0.25)
  Top 0.203: v15.75,21.08 15.62,21.21 12.58,21.21 U3.10
  Bottom 0.203: JP6.11 21.29,12.75 21.29,18.64 21.26,18.67 21.26,20.04 21.03,20.27 20.37,20.27 19.94,20.7 17.35,20.7 16.97,20.32 16.51,20.32 v15.75,21.08
MOSI1  (via drill 0.25)
  Top 0.203: v34.04,21.08 33.91,21.21 30.87,21.21 U4.10
  Bottom 0.203: JP3.11 39.57,12.75 39.57,18.64 39.55,18.67 39.55,20.04 39.32,20.27 38.66,20.27 38.23,20.7 35.64,20.7 35.26,20.32 34.8,20.32 v34.04,21.08
MOSI2  (via drill 0.25)
  Top 0.203: v52.32,21.08 52.2,21.21 49.15,21.21 U6.10
  Bottom 0.203: JP9.11 57.86,12.75 57.86,18.64 57.84,18.67 57.84,20.04 57.61,20.27 56.95,20.27 56.52,20.7 53.92,20.7 53.54,20.32 53.09,20.32 v52.32,21.08
MOSI3  (via drill 0.25)
  Top 0.203: v70.61,21.08 70.48,21.21 67.44,21.21 U8.10
  Bottom 0.203: JP13.11 76.15,12.75 76.15,18.64 76.12,18.67 76.12,20.04 75.89,20.27 75.23,20.27 74.8,20.7 72.21,20.7 71.83,20.32 71.37,20.32 v70.61,21.08
MOSI4  (via drill 0.25)
  Top 0.203: v88.9,21.08 88.77,21.21 85.73,21.21 U10.10
  Bottom 0.203: JP17.11 94.44,12.75 94.44,18.64 94.41,18.67 94.41,20.04 94.18,20.27 93.52,20.27 93.09,20.7 90.5,20.7 90.12,20.32 89.66,20.32 v88.9,21.08
MOSI5  (via drill 0.25)
  Top 0.203: v107.19,21.08 107.06,21.21 104.02,21.21 U12.10
  Bottom 0.203: JP21.11 112.72,12.75 112.72,18.64 112.7,18.67 112.7,20.04 112.47,20.27 111.81,20.27 111.38,20.7 108.79,20.7 108.41,20.32 107.95,20.32 v107.19,21.08
MOSI6  (via drill 0.25)
  Top 0.203: v15.75,57.91 15.62,58.04 12.58,58.04 U14.10
  Bottom 0.203: JP25.11 21.29,49.58 21.29,55.47 21.26,55.5 21.26,56.87 21.03,57.1 20.37,57.1 19.94,57.53 17.35,57.53 16.97,57.15 16.51,57.15 v15.75,57.91
MOSI7  (via drill 0.25)
  Top 0.203: v34.04,57.91 33.91,58.04 30.87,58.04 U16.10
  Bottom 0.203: JP29.11 39.57,49.58 39.57,55.47 39.55,55.5 39.55,56.87 39.32,57.1 38.66,57.1 38.23,57.53 35.64,57.53 35.26,57.15 34.8,57.15 v34.04,57.91
MOSI8  (via drill 0.25)
  Top 0.203: v52.32,57.91 52.2,58.04 49.15,58.04 U18.10
  Bottom 0.203: JP33.11 57.86,49.58 57.86,55.47 57.84,55.5 57.84,56.87 57.61,57.1 56.95,57.1 56.52,57.53 53.92,57.53 53.54,57.15 53.09,57.15 v52.32,57.91
MOSI9  (via drill 0.25)
  Top 0.203: v70.61,57.91 70.48,58.04 67.44,58.04 U20.10
  Bottom 0.203: JP37.11 76.15,49.58 76.15,55.47 76.12,55.5 76.12,56.87 75.89,57.1 75.23,57.1 74.8,57.53 72.21,57.53 71.83,57.15 71.37,57.15 v70.61,57.91
MOSI10  (via drill 0.25)
  Top 0.203: v88.9,57.91 88.77,58.04 85.73,58.04 U22.10
  Bottom 0.203: JP41.11 94.44,49.58 94.44,55.47 94.41,55.5 94.41,56.87 94.18,57.1 93.52,57.1 93.09,57.53 90.5,57.53 90.12,57.15 89.66,57.15 v88.9,57.91
MOSI11  (via drill 0.25)
  Top 0.203: v107.19,57.91 107.06,58.04 104.02,58.04 U24.10
  Bottom 0.203: JP45.11 112.72,49.58 112.72,55.47 112.7,55.5 112.7,56.87 112.47,57.1 111.81,57.1 111.38,57.53 108.79,57.53 108.41,57.15 107.95,57.15 v107.19,57.91
MOSI12  (via drill 0.25)
  Top 0.203: v15.75,94.74 15.62,94.87 12.58,94.87 U26.10
  Bottom 0.203: JP49.11 21.29,86.41 21.29,92.3 21.26,92.33 21.26,93.7 21.03,93.93 20.37,93.93 19.94,94.36 17.35,94.36 16.97,93.98 16.51,93.98 v15.75,94.74
MOSI13  (via drill 0.25)
  Top 0.203: v34.04,94.74 33.91,94.87 30.87,94.87 U28.10
  Bottom 0.203: JP53.11 39.57,86.41 39.57,92.3 39.55,92.33 39.55,93.7 39.32,93.93 38.66,93.93 38.23,94.36 35.64,94.36 35.26,93.98 34.8,93.98 v34.04,94.74
MOSI14  (via drill 0.25)
  Top 0.203: v52.32,94.74 52.2,94.87 49.15,94.87 U30.10
  Bottom 0.203: JP57.11 57.86,86.41 57.86,92.3 57.84,92.33 57.84,93.7 57.61,93.93 56.95,93.93 56.52,94.36 53.92,94.36 53.54,93.98 53.09,93.98 v52.32,94.74
MOSI15  (via drill 0.25)
  Top 0.203: v70.61,94.74 70.48,94.87 67.44,94.87 U32.10
  Bottom 0.203: JP61.11 76.15,86.41 76.15,92.3 76.12,92.33 76.12,93.7 75.89,93.93 75.23,93.93 74.8,94.36 72.21,94.36 71.83,93.98 71.37,93.98 v70.61,94.74
MOSI16  (via drill 0.25)
  Top 0.203: v88.9,94.74 88.77,94.87 85.73,94.87 U34.10
  Bottom 0.203: JP65.11 94.44,86.41 94.44,92.3 94.41,92.33 94.41,93.7 94.18,93.93 93.52,93.93 93.09,94.36 90.5,94.36 90.12,93.98 89.66,93.98 v88.9,94.74
MOSI17  (via drill 0.25)
  Top 0.203: v107.19,94.74 107.06,94.87 104.02,94.87 U36.10
  Bottom 0.203: JP69.11 112.72,86.41 112.72,92.3 112.7,92.33 112.7,93.7 112.47,93.93 111.81,93.93 111.38,94.36 108.79,94.36 108.41,93.98 107.95,93.98 v107.19,94.74
N$1
  Top 0.203: Y1.1 14.03,7.87 15.24,9.08 15.24,11.14 C4.1 14.69,13.31 13.91,14.1 13.21,14.1 12.55,14.76 12.55,15 12.18,15.37 12.18,16.36 11.71,16.84 11.71,17.76 | 12.69,18.47 12.57,18.34 12.29,18.34 11.71,17.76 | 11.71,17.76
N$2
  Top 0.203: Y1.3 18.38,10.95 C2.1 17.53,12.53 15.57,12.53 15.19,12.9 15.19,13.47 14.14,14.52 13.41,14.52 12.95,14.98 12.95,15.23 12.6,15.59 12.6,16.5 12.11,16.99 12.11,17.56 12.49,17.94 12.86,17.94 13.04,18.12
N$3
  Top 0.203: F1.2 14.35,32.76 14.6,33.01 D2.2 13.69,34.33 13.69,35.46 13.46,35.69 13.21,35.69 11.56,37.34 9.65,37.34 9.14,37.85 8.76,37.85 8.54,38.07 SJ1.1
N$4
  Top 0.203: C5.2 10.88,24.99 11.72,24.16 12.42,24.16 U3.6
N$5
  Top 0.203: R4.2 D1.C
N$6
  Top 0.203: X1.D-1 16.4,34.81 16.64,34.57 18.5,34.57 18.71,34.77 R7.2
N$7
  Top 0.203: R6.2 D3.C
N$8
  Top 0.203: X1.D+1 15.75,34.59 16.15,34.19 17.65,34.19 18.5,33.34 R5.2
N$9
  Top 0.203: R1.1 29.46,33.26 LED2.A
N$10
  Top 0.203: Y2.1 32.31,7.87 33.53,9.08 33.53,11.14 C15.1 32.98,13.31 32.19,14.1 31.5,14.1 30.84,14.76 30.84,15 30.47,15.37 30.47,16.36 30,16.84 30,17.76 | 30.98,18.47 30.86,18.34 30.58,18.34 30,17.76 | 30,17.76
N$11
  Top 0.203: Y2.3 36.66,10.95 C14.1 35.82,12.53 33.86,12.53 33.48,12.9 33.48,13.47 32.43,14.52 31.7,14.52 31.24,14.98 31.24,15.23 30.89,15.59 30.89,16.5 30.4,16.99 30.4,17.56 30.78,17.94 31.15,17.94 31.33,18.12
N$12
  Top 0.203: C16.2 29.17,24.99 30.01,24.16 30.71,24.16 U4.6
N$13
  Top 0.203: X2.D-1 34.69,34.81 34.92,34.57 36.79,34.57 37,34.77 R12.2
N$14
  Top 0.203: X2.D+1 34.04,34.59 34.44,34.19 35.94,34.19 36.78,33.34 R10.2
N$15
  Top 0.203: F2.2 32.64,32.76 32.89,33.01 D6.2 31.98,34.33 31.98,35.46 31.75,35.69 31.5,35.69 29.84,37.34 27.94,37.34 27.43,37.85 27.05,37.85 26.83,38.07 SJ2.1
N$16
  Top 0.203: R9.2 D5.C
N$17
  Top 0.203: R8.2 D4.C
N$18
  Top 0.203: R13.1 47.75,33.26 LED3.A
N$19
  Top 0.203: Y3.1 50.6,7.87 51.82,9.08 51.82,11.14 C25.1 51.27,13.31 50.48,14.1 49.79,14.1 49.12,14.76 49.12,15 48.76,15.37 48.76,16.36 48.28,16.84 48.28,17.76 | 49.27,18.47 49.14,18.34 48.87,18.34 48.28,17.76 | 48.28,17.76
N$20
  Top 0.203: Y3.3 54.95,10.95 C24.1 54.11,12.53 52.14,12.53 51.77,12.9 51.77,13.47 50.72,14.52 49.98,14.52 49.53,14.98 49.53,15.23 49.17,15.59 49.17,16.5 48.69,16.99 48.69,17.56 49.06,17.94 49.44,17.94 49.62,18.12
N$21
  Top 0.203: C26.2 47.46,24.99 48.3,24.16 48.99,24.16 U6.6
N$22
  Top 0.203: X3.D-1 52.97,34.81 53.21,34.57 55.08,34.57 55.28,34.77 R18.2
N$23
  Top 0.203: X3.D+1 52.32,34.59 52.73,34.19 54.23,34.19 55.07,33.34 R17.2
N$24
  Top 0.203: F3.2 50.92,32.76 51.17,33.01 D9.2 50.27,34.33 50.27,35.46 50.04,35.69 49.78,35.69 48.13,37.34 46.23,37.34 45.72,37.85 45.34,37.85 45.12,38.07 SJ3.1
N$25
  Top 0.203: R16.2 D8.C
N$26
  Top 0.203: R15.2 D7.C
N$27
  Top 0.203: R19.1 66.04,33.26 LED4.A
N$28
  Top 0.203: Y4.1 68.89,7.87 70.1,9.08 70.1,11.14 C34.1 69.56,13.31 68.77,14.1 68.08,14.1 67.41,14.76 67.41,15 67.04,15.37 67.04,16.36 66.57,16.84 66.57,17.76 | 67.56,18.47 67.43,18.34 67.16,18.34 66.57,17.76 | 66.57,17.76
N$29
  Top 0.203: Y4.3 73.24,10.95 C33.1 72.4,12.53 70.43,12.53 70.06,12.9 70.06,13.47 69.01,14.52 68.27,14.52 67.82,14.98 67.82,15.23 67.46,15.59 67.46,16.5 66.97,16.99 66.97,17.56 67.35,17.94 67.73,17.94 67.9,18.12
N$30
  Top 0.203: C35.2 65.75,24.99 66.58,24.16 67.28,24.16 U8.6
N$31
  Top 0.203: X4.D-1 71.26,34.81 71.5,34.57 73.37,34.57 73.57,34.77 R24.2
N$32
  Top 0.203: X4.D+1 70.61,34.59 71.02,34.19 72.52,34.19 73.36,33.34 R23.2
N$33
  Top 0.203: F4.2 69.21,32.76 69.46,33.01 D12.2 68.56,34.33 68.56,35.46 68.33,35.69 68.07,35.69 66.42,37.34 64.52,37.34 64.01,37.85 63.63,37.85 63.4,38.07 SJ4.1
N$34
  Top 0.203: R22.2 D11.C
N$35
  Top 0.203: R21.2 D10.C
N$36
  Top 0.203: R25.1 84.33,33.26 LED5.A
N$37
  Top 0.203: Y5.1 87.18,7.87 88.39,9.08 88.39,11.14 C43.1 87.84,13.31 87.06,14.1 86.36,14.1 85.7,14.76 85.7,15 85.33,15.37 85.33,16.36 84.86,16.84 84.86,17.76 | 85.84,18.47 85.72,18.34 85.45,18.34 84.86,17.76 | 84.86,17.76
N$38
  Top 0.203: R11.1 11.18,33.26 LED1.A
N$39
  Top 0.203: Y5.3 91.53,10.95 C42.1 90.69,12.53 88.72,12.53 88.35,12.9 88.35,13.47 87.3,14.52 86.56,14.52 86.11,14.98 86.11,15.23 85.75,15.59 85.75,16.5 85.26,16.99 85.26,17.56 85.64,17.94 86.02,17.94 86.19,18.12
N$40
  Top 0.203: C44.2 84.04,24.99 84.87,24.16 85.57,24.16 U10.6
N$41
  Top 0.203: X5.D-1 89.55,34.81 89.79,34.57 91.66,34.57 91.86,34.77 R30.2
N$42
  Top 0.203: X5.D+1 88.9,34.59 89.31,34.19 90.81,34.19 91.65,33.34 R29.2
N$43
  Top 0.203: F5.2 87.5,32.76 87.75,33.01 D15.2 86.84,34.33 86.84,35.46 86.61,35.69 86.36,35.69 84.71,37.34 82.8,37.34 82.3,37.85 81.92,37.85 81.69,38.07 SJ5.1
N$44
  Top 0.203: R28.2 D14.C
N$45
  Top 0.203: R27.2 D13.C
N$46
  Top 0.203: R31.1 102.61,33.26 LED6.A
N$47
  Top 0.203: Y6.1 105.47,7.87 106.68,9.08 106.68,11.14 C52.1 106.13,13.31 105.35,14.1 104.65,14.1 103.99,14.76 103.99,15 103.62,15.37 103.62,16.36 103.15,16.84 103.15,17.76 | 104.13,18.47 104.01,18.34 103.73,18.34 103.15,17.76 | 103.15,17.76
N$48
  Top 0.203: Y6.3 109.82,10.95 C51.1 108.97,12.53 107.01,12.53 106.63,12.9 106.63,13.47 105.58,14.52 104.85,14.52 104.39,14.98 104.39,15.23 104.04,15.59 104.04,16.5 103.55,16.99 103.55,17.56 103.93,17.94 104.3,17.94 104.48,18.12
N$49
  Top 0.203: C53.2 102.32,24.99 103.16,24.16 103.86,24.16 U12.6
N$50
  Top 0.203: X6.D-1 107.84,34.81 108.08,34.57 109.94,34.57 110.15,34.77 R36.2
N$51
  Top 0.203: X6.D+1 107.19,34.59 107.59,34.19 109.09,34.19 109.94,33.34 R35.2
N$52
  Top 0.203: F6.2 105.79,32.76 106.04,33.01 D18.2 105.13,34.33 105.13,35.46 104.9,35.69 104.65,35.69 103,37.34 101.09,37.34 100.58,37.85 100.2,37.85 99.98,38.07 SJ6.1
N$53
  Top 0.203: R34.2 D17.C
N$54
  Top 0.203: R33.2 D16.C
N$55
  Top 0.203: R37.1 11.18,70.09 LED7.A
N$56
  Top 0.203: Y7.1 14.03,44.7 15.24,45.91 15.24,47.97 C61.1 14.69,50.14 13.91,50.93 13.21,50.93 12.55,51.59 12.55,51.83 12.18,52.2 12.18,53.19 11.71,53.66 11.71,54.59 | 12.69,55.3 12.57,55.17 12.29,55.17 11.71,54.59 | 11.71,54.59
N$57
  Top 0.203: Y7.3 18.38,47.77 C60.1 17.53,49.36 15.57,49.36 15.19,49.73 15.19,50.3 14.14,51.35 13.41,51.35 12.95,51.81 12.95,52.06 12.6,52.42 12.6,53.33 12.11,53.82 12.11,54.39 12.49,54.77 12.86,54.77 13.04,54.95
N$58
  Top 0.203: C62.2 10.88,61.82 11.72,60.99 12.42,60.99 U14.6
N$59
  Top 0.203: X7.D-1 16.4,71.64 16.64,71.4 18.5,71.4 18.71,71.6 R42.2
N$60
  Top 0.203: X7.D+1 15.75,71.42 16.15,71.02 17.65,71.02 18.5,70.17 R41.2
N$61
  Top 0.203: F7.2 14.35,69.59 14.6,69.84 D21.2 13.69,71.16 13.69,72.29 13.46,72.52 13.21,72.52 11.56,74.17 9.65,74.17 9.14,74.68 8.76,74.68 8.54,74.9 SJ7.1
N$62
  Top 0.203: R40.2 D20.C
N$63
  Top 0.203: R39.2 D19.C
N$64
  Top 0.203: R43.1 29.46,70.09 LED8.A
N$65
  Top 0.203: Y8.1 32.31,44.7 33.53,45.91 33.53,47.97 C70.1 32.98,50.14 32.19,50.93 31.5,50.93 30.84,51.59 30.84,51.83 30.47,52.2 30.47,53.19 30,53.66 30,54.59 | 30.98,55.3 30.86,55.17 30.58,55.17 30,54.59 | 30,54.59
N$66
  Top 0.203: Y8.3 36.66,47.77 C69.1 35.82,49.36 33.86,49.36 33.48,49.73 33.48,50.3 32.43,51.35 31.7,51.35 31.24,51.81 31.24,52.06 30.89,52.42 30.89,53.33 30.4,53.82 30.4,54.39 30.78,54.77 31.15,54.77 31.33,54.95
N$67
  Top 0.203: C71.2 29.17,61.82 30.01,60.99 30.71,60.99 U16.6
N$68
  Top 0.203: X8.D-1 34.69,71.64 34.92,71.4 36.79,71.4 37,71.6 R48.2
N$69
  Top 0.203: X8.D+1 34.04,71.42 34.44,71.02 35.94,71.02 36.78,70.17 R47.2
N$70
  Top 0.203: F8.2 32.64,69.59 32.89,69.84 D24.2 31.98,71.16 31.98,72.29 31.75,72.52 31.5,72.52 29.84,74.17 27.94,74.17 27.43,74.68 27.05,74.68 26.83,74.9 SJ8.1
N$71
  Top 0.203: R46.2 D23.C
N$72
  Top 0.203: R45.2 D22.C
N$73
  Top 0.203: R49.1 47.75,70.09 LED9.A
N$74
  Top 0.203: Y9.1 50.6,44.7 51.82,45.91 51.82,47.97 C79.1 51.27,50.14 50.48,50.93 49.79,50.93 49.12,51.59 49.12,51.83 48.76,52.2 48.76,53.19 48.28,53.66 48.28,54.59 | 49.27,55.3 49.14,55.17 48.87,55.17 48.28,54.59 | 48.28,54.59
N$75
  Top 0.203: Y9.3 54.95,47.77 C78.1 54.11,49.36 52.14,49.36 51.77,49.73 51.77,50.3 50.72,51.35 49.98,51.35 49.53,51.81 49.53,52.06 49.17,52.42 49.17,53.33 48.69,53.82 48.69,54.39 49.06,54.77 49.44,54.77 49.62,54.95
N$76
  Top 0.203: C80.2 47.46,61.82 48.3,60.99 48.99,60.99 U18.6
N$77
  Top 0.203: X9.D-1 52.97,71.64 53.21,71.4 55.08,71.4 55.28,71.6 R54.2
N$78
  Top 0.203: X9.D+1 52.32,71.42 52.73,71.02 54.23,71.02 55.07,70.17 R53.2
N$79
  Top 0.203: F9.2 50.92,69.59 51.17,69.84 D27.2 50.27,71.16 50.27,72.29 50.04,72.52 49.78,72.52 48.13,74.17 46.23,74.17 45.72,74.68 45.34,74.68 45.12,74.9 SJ9.1
N$80
  Top 0.203: R52.2 D26.C
N$81
  Top 0.203: R51.2 D25.C
N$82
  Top 0.203: R55.1 66.04,70.09 LED10.A
N$83
  Top 0.203: Y10.1 68.89,44.7 70.1,45.91 70.1,47.97 C88.1 69.56,50.14 68.77,50.93 68.08,50.93 67.41,51.59 67.41,51.83 67.04,52.2 67.04,53.19 66.57,53.66 66.57,54.59 | 67.56,55.3 67.43,55.17 67.16,55.17 66.57,54.59 | 66.57,54.59
N$84
  Top 0.203: Y10.3 73.24,47.77 C87.1 72.4,49.36 70.43,49.36 70.06,49.73 70.06,50.3 69.01,51.35 68.27,51.35 67.82,51.81 67.82,52.06 67.46,52.42 67.46,53.33 66.97,53.82 66.97,54.39 67.35,54.77 67.73,54.77 67.9,54.95
N$85
  Top 0.203: C89.2 65.75,61.82 66.58,60.99 67.28,60.99 U20.6
N$86
  Top 0.203: X10.D-1 71.26,71.64 71.5,71.4 73.37,71.4 73.57,71.6 R60.2
N$87
  Top 0.203: X10.D+1 70.61,71.42 71.02,71.02 72.52,71.02 73.36,70.17 R59.2
N$88
  Top 0.203: F10.2 69.21,69.59 69.46,69.84 D30.2 68.56,71.16 68.56,72.29 68.33,72.52 68.07,72.52 66.42,74.17 64.52,74.17 64.01,74.68 63.63,74.68 63.4,74.9 SJ10.1
N$89
  Top 0.203: R58.2 D29.C
N$90
  Top 0.203: R57.2 D28.C
N$91
  Top 0.203: R61.1 84.33,70.09 LED11.A
N$92
  Top 0.203: Y11.1 87.18,44.7 88.39,45.91 88.39,47.97 C97.1 87.84,50.14 87.06,50.93 86.36,50.93 85.7,51.59 85.7,51.83 85.33,52.2 85.33,53.19 84.86,53.66 84.86,54.59 | 85.84,55.3 85.72,55.17 85.45,55.17 84.86,54.59 | 84.86,54.59
N$93
  Top 0.203: Y11.3 91.53,47.77 C96.1 90.69,49.36 88.72,49.36 88.35,49.73 88.35,50.3 87.3,51.35 86.56,51.35 86.11,51.81 86.11,52.06 85.75,52.42 85.75,53.33 85.26,53.82 85.26,54.39 85.64,54.77 86.02,54.77 86.19,54.95
N$94
  Top 0.203: C98.2 84.04,61.82 84.87,60.99 85.57,60.99 U22.6
N$95
  Top 0.203: X11.D-1 89.55,71.64 89.79,71.4 91.66,71.4 91.86,71.6 R66.2
N$96
  Top 0.203: X11.D+1 88.9,71.42 89.31,71.02 90.81,71.02 91.65,70.17 R65.2
N$97
  Top 0.203: F11.2 87.5,69.59 87.75,69.84 D33.2 86.84,71.16 86.84,72.29 86.61,72.52 86.36,72.52 84.71,74.17 82.8,74.17 82.3,74.68 81.92,74.68 81.69,74.9 SJ11.1
N$98
  Top 0.203: R64.2 D32.C
N$99
  Top 0.203: R63.2 D31.C
N$100
  Top 0.203: R67.1 102.61,70.09 LED12.A
N$101
  Top 0.203: Y12.1 105.47,44.7 106.68,45.91 106.68,47.97 C106.1 106.13,50.14 105.35,50.93 104.65,50.93 103.99,51.59 103.99,51.83 103.62,52.2 103.62,53.19 103.15,53.66 103.15,54.59 | 104.13,55.3 104.01,55.17 103.73,55.17 103.15,54.59 | 103.15,54.59
N$102
  Top 0.203: Y12.3 109.82,47.77 C105.1 108.97,49.36 107.01,49.36 106.63,49.73 106.63,50.3 105.58,51.35 104.85,51.35 104.39,51.81 104.39,52.06 104.04,52.42 104.04,53.33 103.55,53.82 103.55,54.39 103.93,54.77 104.3,54.77 104.48,54.95
N$103
  Top 0.203: C107.2 102.32,61.82 103.16,60.99 103.86,60.99 U24.6
N$104
  Top 0.203: X12.D-1 107.84,71.64 108.08,71.4 109.94,71.4 110.15,71.6 R72.2
N$105
  Top 0.203: X12.D+1 107.19,71.42 107.59,71.02 109.09,71.02 109.94,70.17 R71.2
N$106
  Top 0.203: F12.2 105.79,69.59 106.04,69.84 D36.2 105.13,71.16 105.13,72.29 104.9,72.52 104.65,72.52 103,74.17 101.09,74.17 100.58,74.68 100.2,74.68 99.98,74.9 SJ12.1
N$107
  Top 0.203: R70.2 D35.C
N$108
  Top 0.203: R69.2 D34.C
N$109
  Top 0.203: R73.1 11.18,106.92 LED13.A
N$110
  Top 0.203: Y13.1 14.03,81.53 15.24,82.74 15.24,84.8 C115.1 14.69,86.97 13.91,87.76 13.21,87.76 12.55,88.42 12.55,88.66 12.18,89.03 12.18,90.02 11.71,90.5 11.71,91.42 | 12.69,92.13 12.57,92 12.29,92 11.71,91.42 | 11.71,91.42
N$111
  Top 0.203: Y13.3 18.38,84.61 C114.1 17.53,86.19 15.57,86.19 15.19,86.56 15.19,87.13 14.14,88.18 13.41,88.18 12.95,88.64 12.95,88.89 12.6,89.25 12.6,90.16 12.11,90.65 12.11,91.22 12.49,91.6 12.86,91.6 13.04,91.78
N$112
  Top 0.203: C116.2 10.88,98.65 11.72,97.82 12.42,97.82 U26.6
N$113
  Top 0.203: X13.D-1 16.4,108.47 16.64,108.23 18.5,108.23 18.71,108.43 R78.2
N$114
  Top 0.203: X13.D+1 15.75,108.25 16.15,107.85 17.65,107.85 18.5,107 R77.2
N$115
  Top 0.203: F13.2 14.35,106.42 14.6,106.67 D39.2 13.69,107.99 13.69,109.12 13.46,109.35 13.21,109.35 11.56,111 9.65,111 9.14,111.51 8.76,111.51 8.54,111.73 SJ13.1
N$116
  Top 0.203: R76.2 D38.C
N$117
  Top 0.203: R75.2 D37.C
N$118
  Top 0.203: R79.1 29.46,106.92 LED14.A
N$119
  Top 0.203: Y14.1 32.31,81.53 33.53,82.74 33.53,84.8 C124.1 32.98,86.97 32.19,87.76 31.5,87.76 30.84,88.42 30.84,88.66 30.47,89.03 30.47,90.02 30,90.5 30,91.42 | 30.98,92.13 30.86,92 30.58,92 30,91.42 | 30,91.42
N$120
